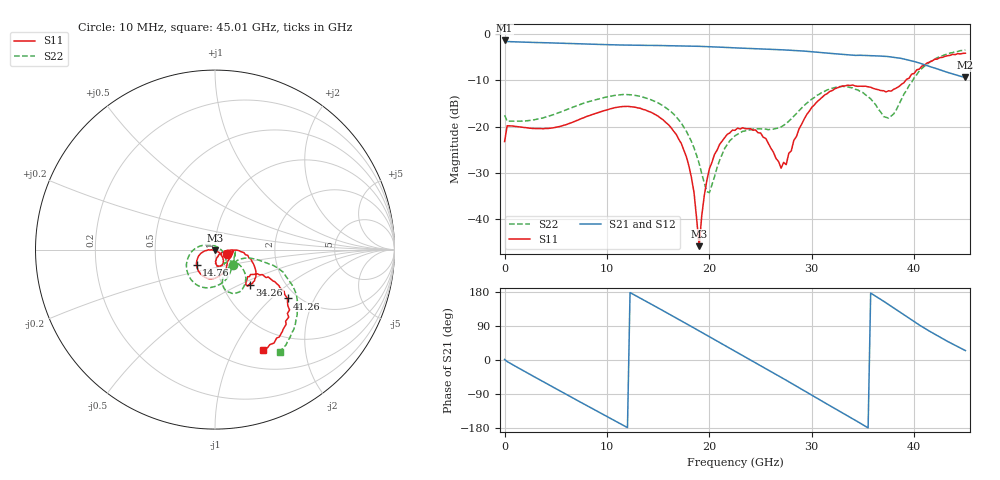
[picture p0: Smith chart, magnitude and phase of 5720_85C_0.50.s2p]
! Device:  ADRF5720
! Description: 0.5dB LSB GaAs MMIC 6-bit Digital Attenuator
! Frequency:  0.000009 -  40 GHz
! Ports:
!	RF1	= Port 1
!	RF2	= Port 2
! Vdd:  3.3 Volt
! Vss:  -3.3 Volt
! Control:  0/3.3 Volt
! State:  0.50 dB attenuation
! Data:  The device was measured using G-S-G Probes on a matrix board.
!  Data was collected using an calibrated 4 port network analyzer.
!  The reference plane for this measurement is at the launchers.
! Note:  Analog Devices supplies this data as a sample of measured data
!  for this product.  Your particular data for this product may vary.
!  Data was taken at 85 degrees C.
!  Analog Devices reserves the right to change this data at anytime.
# GHZ S DB R 45.0
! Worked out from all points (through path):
!   181 points, 10 MHz to 45.01 GHz, reference 45 ohm
!   highest |S21| = -1.36 dB at 10 MHz (marker M1); lowest = -9.4 dB at 45.01 GHz (marker M2)
!   group delay of S21, straight-line fit = 42.9 ps
!   lowest |S11| = -45.9 dB at 19.01 GHz (marker M3), VSWR 1.01, Z = 44.8 - j0.426 ohm
!   |S11| at or under -10 dB: start of sweep to 39.18 GHz
!   |S22| runs from -34.3 to -3.4 dB; largest |S21 - S12| = 0.004
!   S11 on the Smith chart (normalised r, x): 10 MHz: 1.14, -0.05; 14.76 GHz: 0.80, -0.14; 34.26 GHz: 1.34, -0.57; 41.26 GHz: 1.78, -1.27; 45.01 GHz: 0.72, -1.32
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0.01  -23.24 -20.0  -1.36 1.4  -1.35 1.5  -17.55 -39.7
0.26  -19.83 -4.8  -1.59 -4.1  -1.59 -4.0  -18.84 -4.1
4.01  -20.41 -39.5  -1.86 -60.7  -1.84 -60.7  -17.96 -39.2
6.01  -19.60 -50.1  -1.99 -90.4  -1.97 -90.3  -16.38 -55.7
7.76  -18.08 -61.2  -2.11 -116.2  -2.10 -116.2  -14.92 -70.9
11.26  -15.74 -96.6  -2.34 -167.5  -2.32 -167.4  -13.13 -107.0
14.76  -17.46 -140.1  -2.45 140.9  -2.43 141.1  -14.63 -149.0
15.26  -18.20 -146.3  -2.46 133.5  -2.44 133.6  -15.22 -155.4
17.76  -26.54 -173.8  -2.55 95.8  -2.53 96.0  -21.01 168.2
18.51  -34.34 -175.9  -2.59 84.4  -2.57 84.6  -24.63 152.1
19.01  -45.90 -110.3  -2.63 76.8  -2.61 76.9  -28.01 136.3
19.51  -34.95 -41.4  -2.67 69.1  -2.65 69.3  -32.20 107.8
20.01  -29.13 -40.2  -2.71 61.5  -2.69 61.7  -34.32 52.7
21.51  -22.38 -51.2  -2.86 38.6  -2.84 38.8  -24.69 -24.9
22.76  -20.34 -65.6  -2.99 19.6  -2.96 19.9  -21.67 -43.1
25.01  -21.40 -84.8  -3.20 -14.6  -3.18 -14.4  -20.50 -57.8
27.01  -29.01 -55.0  -3.38 -45.6  -3.36 -45.3  -20.07 -41.0
30.26  -15.32 -9.5  -3.86 -96.9  -3.84 -96.6  -13.72 -37.2
34.26  -11.23 -45.2  -4.59 -159.1  -4.57 -158.8  -11.93 -70.6
37.76  -12.33 -35.1  -4.94 141.8  -4.92 142.2  -17.73 -34.5
41.26  -6.25 -33.9  -6.79 79.9  -6.77 80.3  -6.50 -24.6
45.01  -4.12 -64.6  -9.38 24.8  -9.35 25.2  -3.41 -57.5
